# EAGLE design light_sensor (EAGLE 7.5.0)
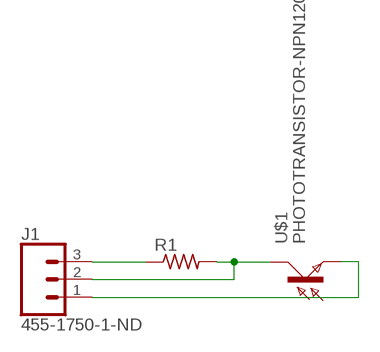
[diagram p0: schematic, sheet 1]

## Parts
J1  455-1750-1-ND  CONN_03  [1X03]
R1  RES-US1206FAB  [R1206FAB]
U$1  PHOTOTRANSISTOR-NPN1206  [OP1206]

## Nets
N$1: J1.2 R1.2 U$1.COLLECTOR(C)
N$3: J1.1 U$1.EMITTER(E)
VCC: J1.3 R1.1

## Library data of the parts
J1 = SparkFun-Connectors:CONN_03: Multi connection point. Often used as Generic Header-pin footprint for 0.1 inch spaced/style header connections On any of the 0.1 inch spaced packages, you can populate with these: Break Away Headers - Straight (PRT-00116) Break Away Male Headers - Right Angle (PRT-00553) Female Headers (PRT-00115)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; PROD_ID: XXX-00000
R1 = fab:RES-US: Resistor (US Symbol)
U$1 = fab:PHOTOTRANSISTOR-NPN

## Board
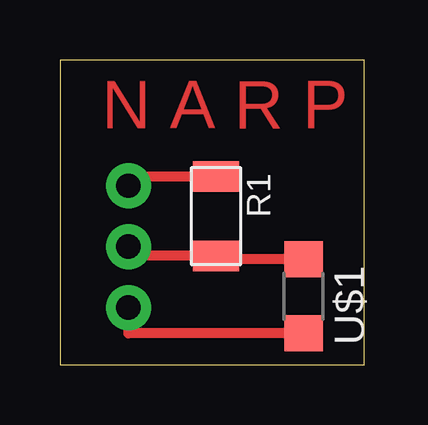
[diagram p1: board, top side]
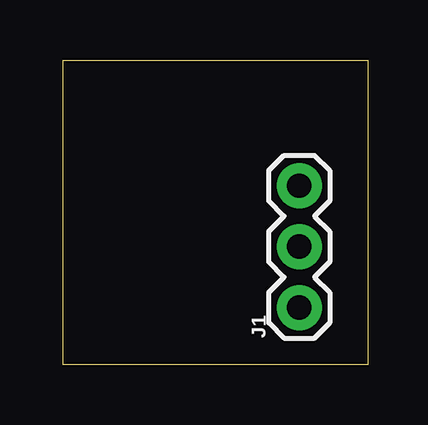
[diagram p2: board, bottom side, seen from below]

Size 12.7 x 12.7 mm. Coordinates in mm from the lower left corner, seen from the top.
Outline: 0,0 12.7,0 12.7,12.7 0,12.7 0,0
Copper layers (1*16): Top 0.035mm / dielectric 1.5mm / Bottom 0.035mm
Design rules "default": minimum track width 10mil, minimum drill 24mil, track to track 8mil, track to pad 8mil, pad to pad 8mil, via to via 8mil, smd to smd 8mil, copper to edge 40mil, drill to drill 8mil, minimum pad ring 10mil, minimum via ring 8mil, stop-mask expansion 4mil, vias tented up to drill 0mil, thermal gap 10mil

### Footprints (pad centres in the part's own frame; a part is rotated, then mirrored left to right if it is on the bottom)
1X03 = drill 1.016 pad 1.88: 1 0,0; 2 2.54,0; 3 5.08,0
R1206FAB = smd 1.27 x 1.905: 1 -1.651,0; 2 1.651,0
OP1206 = smd 1.5 x 1.6: COLLECTOR -1.55,0; EMITTER 1.55,0

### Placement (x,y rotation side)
J1  2.86,2.38 90 bottom
R1  6.51,6.19 270 top
U$1  10.16,2.86 270 top

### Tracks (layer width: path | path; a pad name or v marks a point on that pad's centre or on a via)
N$1
  Top 0.406: U$1.COLLECTOR 6.51,4.41 R1.2 2.86,4.54 J1.2
N$3
  Top 0.406: U$1.EMITTER 2.86,1.31 J1.1
VCC
  Top 0.406: R1.1 2.86,7.84 J1.3

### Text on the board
Top: N A R P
